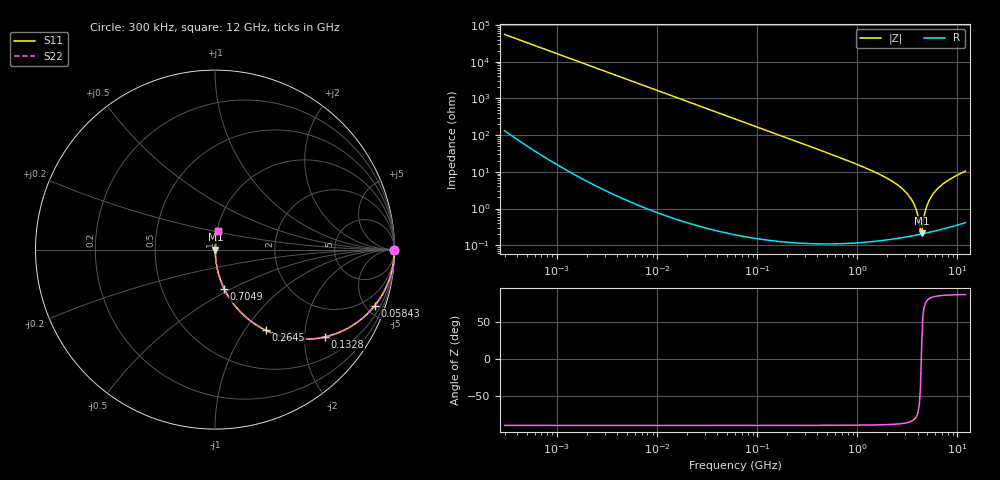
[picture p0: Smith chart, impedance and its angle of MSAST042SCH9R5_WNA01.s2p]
! MSAST042SCH9R5_WNA01  S-PARAMETER MODEL  ( General Type )
! Model Generated by TAIYO YUDEN Corporation (http://www.ty-top.com)
! Version 1.0
! TAIYO YUDEN Control No. 150820
! Copyright(c) 2015 TAIYO YUDEN CO.,LTD. All Rights Reserved.
! Product Description (link to TY-COMPAS)
! https://ds.yuden.co.jp/TYCOMPAS/or/detail?pn=MSAST042SCH9R5BWNA01&u=M
! Products Name : Multilayer Ceramic Capacitors
! Characteristics :
!  Capacitance : 9.5 pF , Rated Voltage : 25V , TCC : CH / C0H
!  Case Size : 0.4 x 0.2 / 0.016 x 0.008 [mm/inch] , Thickness : 0.2 / 0.008 [mm/inch]
!  (Conditions: Temperature = 25 degC , DC Bias Current/Voltage = 0A / 0V)
! External Node Assignments :
!  1  o---| |---o  2
! GND o---------o GND
! Frequency Range : 0.3MHz  -  12000MHz  [ 401 STEP ]
# MHz S RI R 50
! Freq[MHz].  S11 Real  S11 Imag  S21 Real  S21 Imag  S12 Real  S12 Imag  S22 Real  S22 Imag
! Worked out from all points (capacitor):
!   401 points, 300 kHz to 12 GHz, reference 50 ohm
!   read as one part in series: C = 9.53 pF near 316.3 kHz
!   lowest |Z| = 209 mohm at 4.385 GHz (marker M1)
!   series resonance near 4.356 GHz, so ESL is about 140 pH
!   S11 on the Smith chart (normalised r, x): 300 kHz: open; 58.43 MHz: 1.00, -5.72; 132.8 MHz: 1.00, -2.51; 264.5 MHz: 1.00, -1.26; 704.9 MHz: 1.00, -0.46; 12 GHz: 1.01, +0.21
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0.3  1 -0.0018  7.45e-06 0.0018  7.45e-06 0.0018  1 -0.0018
1.769972  0.9999 -0.0106  0.00012 0.0106  0.00012 0.0106  0.9999 -0.0106
10.44266  0.9961 -0.0623  0.00392 0.0623  0.00392 0.0623  0.9961 -0.0623
25.70316  0.9768 -0.1503  0.0232 0.1503  0.0232 0.1503  0.9768 -0.1503
58.43137  0.8908 -0.3115  0.1092 0.3115  0.1092 0.3115  0.8908 -0.3115
60  0.8855 -0.318  0.1145 0.318  0.1145 0.318  0.8855 -0.318
132.8329  0.6121 -0.4867  0.3879 0.4867  0.3879 0.4867  0.6121 -0.4867
264.5085  0.284 -0.45  0.716 0.45  0.716 0.45  0.284 -0.45
353.9943  0.1808 -0.3837  0.8192 0.3837  0.8192 0.3837  0.1808 -0.3837
704.9044  0.0515 -0.2187  0.9485 0.2187  0.9485 0.2187  0.0515 -0.2187
2088.533  0.00519 -0.0612  0.9948 0.0612  0.9948 0.0612  0.00519 -0.0612
2795.104  0.00283 -0.035  0.9972 0.035  0.9972 0.035  0.00283 -0.035
3364.605  0.00215 -0.02  0.9978 0.02  0.9978 0.02  0.00215 -0.02
3841.137  0.00197 -0.0097  0.998 0.0097  0.998 0.0097  0.00197 -0.0097
4158.869  0.00197 -0.0036  0.998 0.0036  0.998 0.0036  0.00197 -0.0036
4270.516  0.00199 -0.00158  0.998 0.00158  0.998 0.00158  0.00199 -0.00158
4385.161  0.00202 0.000532  0.998 -0.000532  0.998 -0.000532  0.00202 0.000532
4502.883  0.00205 0.00297  0.9979 -0.00297  0.9979 -0.00297  0.00205 0.00297
5006.236  0.00234 0.0125  0.9977 -0.0125  0.9977 -0.0125  0.00234 0.0125
5868.704  0.00316 0.0275  0.9968 -0.0275  0.9968 -0.0275  0.00316 0.0275
7648.807  0.00569 0.0529  0.9943 -0.0529  0.9943 -0.0529  0.00569 0.0529
12000  0.0147 0.1026  0.9853 -0.1026  0.9853 -0.1026  0.0147 0.1026
